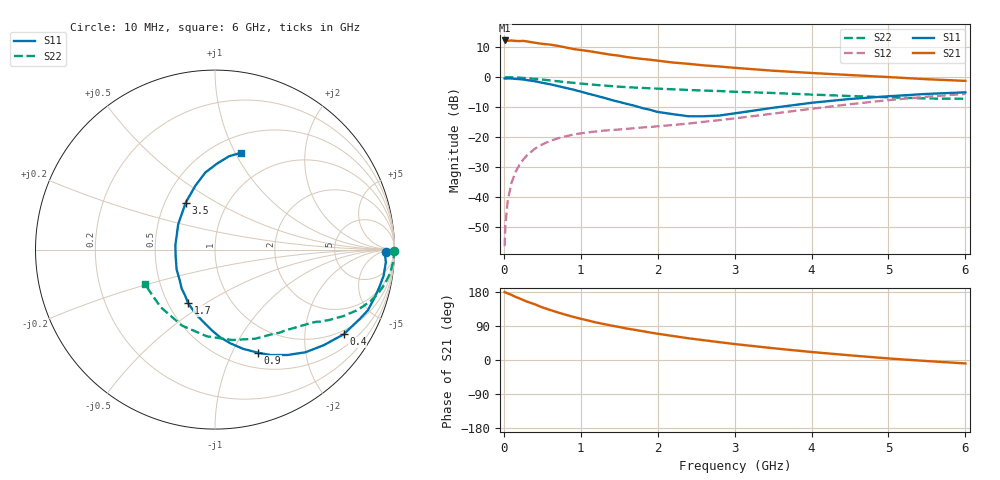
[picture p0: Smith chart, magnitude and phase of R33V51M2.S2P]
! SIEMENS Small Signal Semiconductors
! BFR181
! Si NPN RF Bipolar Junction Transistor in SOT23
! VCE = 3.5 V  IC = 1.2 mA
! Common Emitter S-Parameters:  May  1996
# GHz  S  MA  R  50
!  f  S11  S21  S12  S22
! GHz  MAG  ANG  MAG  ANG  MAG  ANG  MAG  ANG
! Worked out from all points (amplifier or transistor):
!   36 points, 10 MHz to 6 GHz, reference 50 ohm
!   highest |S21| = 12.3 dB at 10 MHz (marker M1)
!   |S21| within 3 dB of that: start of sweep to 944.2 MHz
!   unconditionally stable (mu >= 1): 1.922 GHz to 3.602 GHz
!   at 250 MHz: K = 0.17, MSG = 19.9 dB, |S12| = -27.6 dB
!   at 1.4 GHz: K = 0.82, MSG = 12.6 dB, |S12| = -17.7 dB
!   at 6 GHz: K = 0.87, MSG = 2.2 dB, |S12| = -5.6 dB
!   S11 on the Smith chart (normalised r, x): 10 MHz: 39, -12; 400 MHz: 0.87, -3.11; 900 MHz: 0.67, -1.26; 1.7 GHz: 0.63, -0.42; 3.5 GHz: 0.64, +0.37; 6 GHz: 0.67, +1.06
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0.01  0.9542 -0.8  4.113 179.4  0.0015 91.6  0.9978 -0.4
0.02  0.9475 -1.8  4.071 178.2  0.0033 88.3  0.9881 -0.8
0.05  0.9544 -4.2  4.06 175.9  0.0086 86.5  0.997 -2.0
0.1  0.9509 -8.7  4.108 171.8  0.0172 83.7  0.9946 -4.0
0.15  0.939 -12.9  4.038 166.8  0.0257 81.2  0.9882 -6.2
0.25  0.9162 -21.7  4.043 158.4  0.0417 76.2  0.9732 -9.9
0.3  0.8943 -25.6  3.966 154.2  0.0493 73.9  0.9625 -11.8
0.4  0.858 -33.4  3.77 147.2  0.0633 69.4  0.9411 -15.1
0.5  0.8067 -41.3  3.611 138.9  0.0753 65.0  0.9135 -18.2
0.6  0.7625 -48.6  3.506 132.1  0.0862 61.2  0.8834 -21.0
0.7  0.7132 -55.4  3.344 125.7  0.0948 58.1  0.8551 -23.5
0.9  0.6214 -67.5  2.965 114.0  0.11 53.0  0.8068 -27.3
1.1  0.5295 -80.6  2.734 104.0  0.1199 49.4  0.763 -30.4
1.4  0.4157 -97.7  2.368 90.8  0.1304 47.0  0.7091 -34.5
1.7  0.3334 -116.8  2.089 79.7  0.1404 46.6  0.6714 -37.6
1.9  0.2853 -130.7  1.958 72.6  0.1473 47.1  0.6524 -40.0
2.2  0.2408 -152.6  1.758 63.3  0.1589 48.4  0.6275 -43.5
2.8  0.2286 158.3  1.51 47.1  0.1914 51.5  0.5873 -52.0
3.5  0.3082 122.0  1.283 31.1  0.246 52.2  0.5449 -65.7
4.5  0.4331 97.1  1.086 12.3  0.3537 46.7  0.4851 -95.5
5.5  0.5259 81.4  0.925 -2.8  0.4721 34.2  0.441 -133.5
6  0.559 74.9  0.868 -9.1  0.5256 26.6  0.4359 -153.9
